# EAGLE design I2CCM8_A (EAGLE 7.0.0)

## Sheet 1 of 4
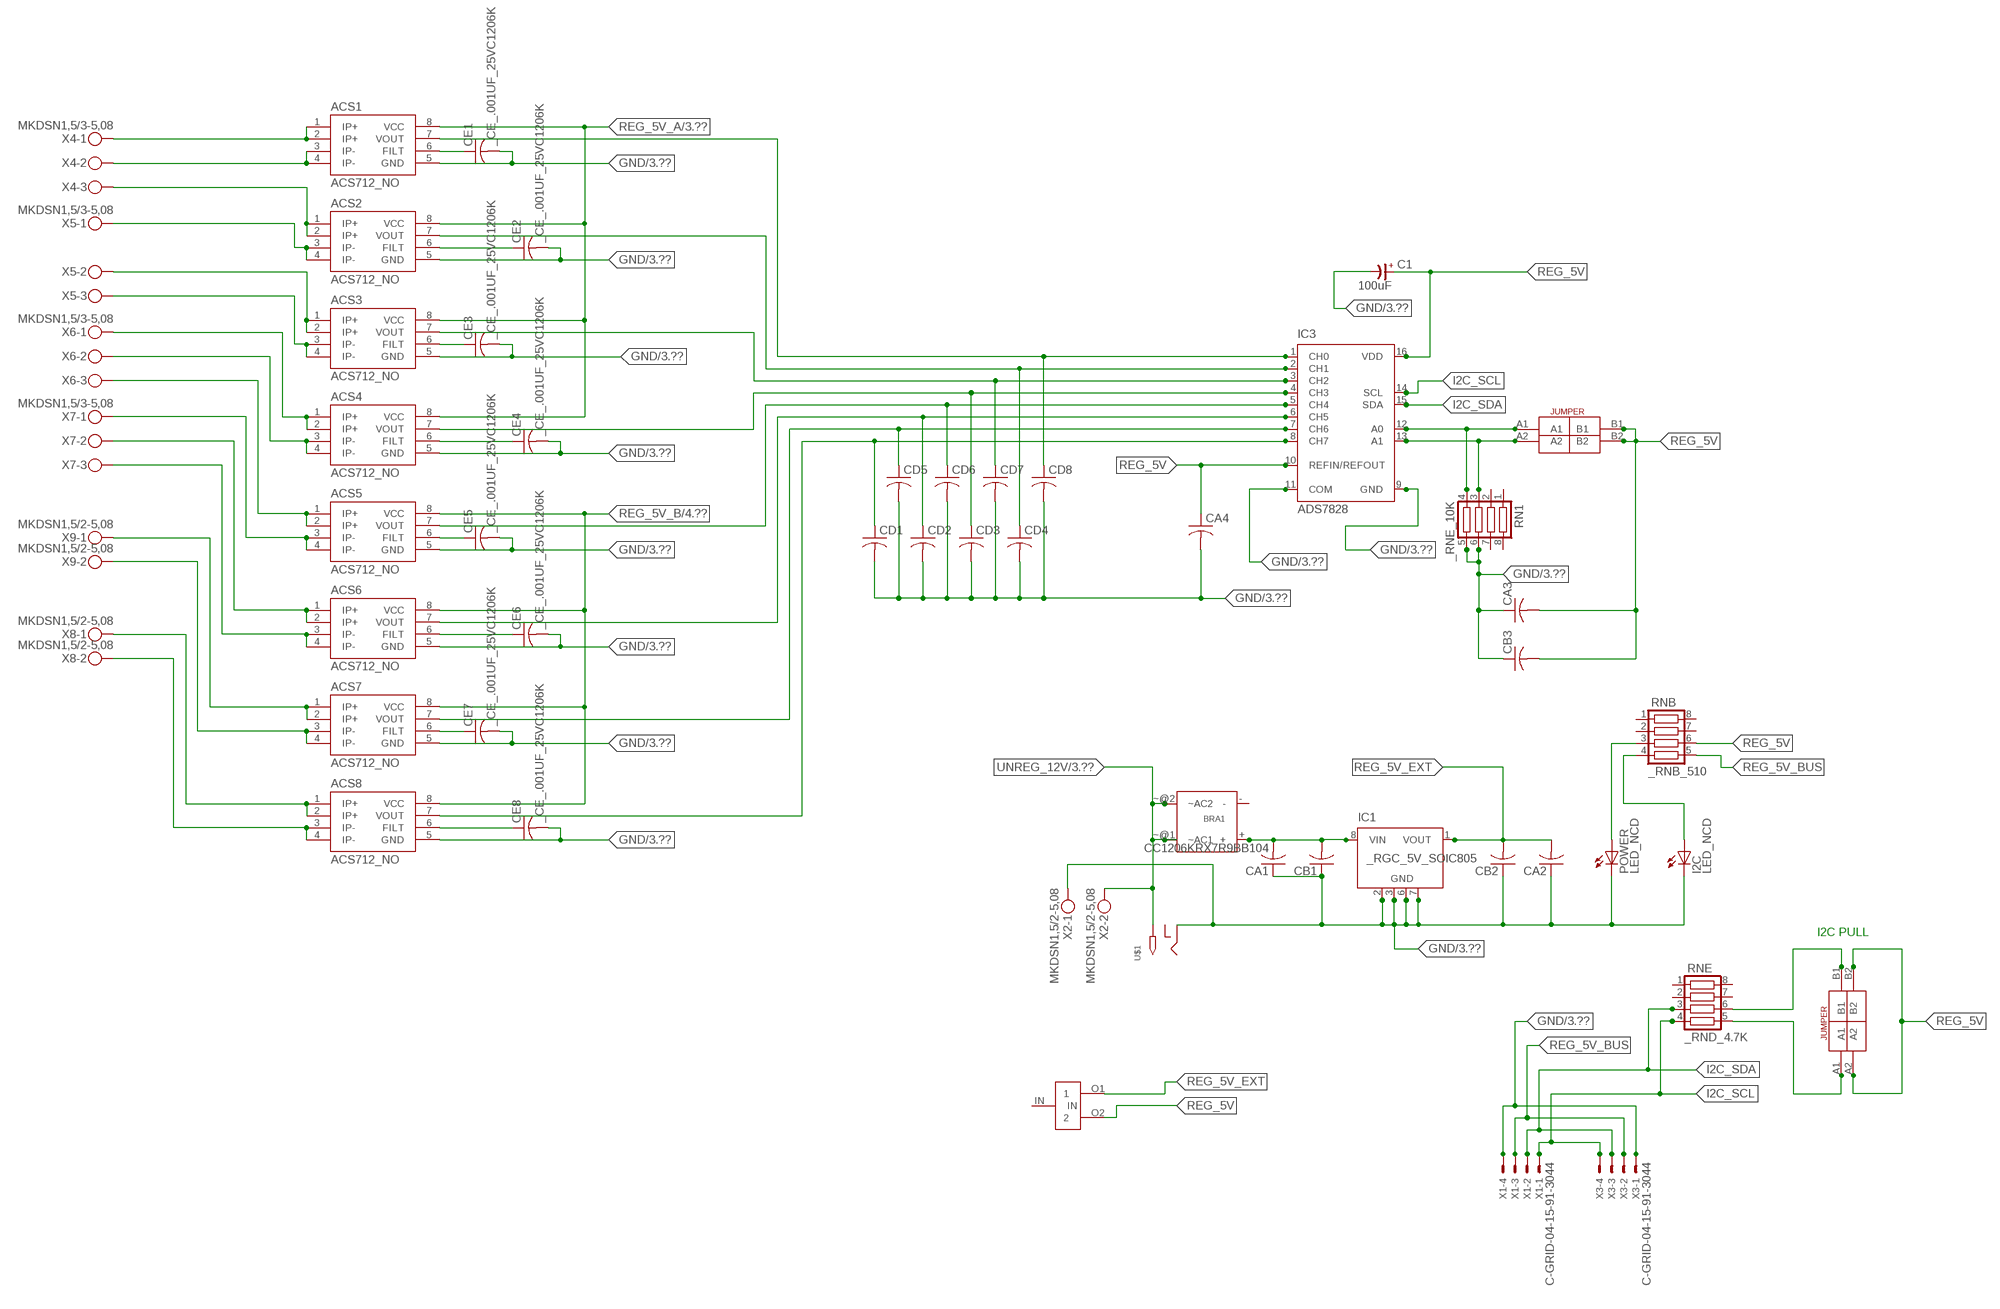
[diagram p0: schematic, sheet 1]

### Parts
ACS1  ACS712_NO  [_MA_DUAL_N-FET]
ACS2  ACS712_NO  [_MA_DUAL_N-FET]
ACS3  ACS712_NO  [_MA_DUAL_N-FET]
ACS4  ACS712_NO  [_MA_DUAL_N-FET]
ACS5  ACS712_NO  [_MA_DUAL_N-FET]
ACS6  ACS712_NO  [_MA_DUAL_N-FET]
ACS7  ACS712_NO  [_MA_DUAL_N-FET]
ACS8  ACS712_NO  [_MA_DUAL_N-FET]
BRA1  MB2S_  [MB2S]
C1  100uF  CP-E-025X060  [E-025X060]
CA1  CC1206KRX7R9BB104  [.1UF]
CA2  CC1206KRX7R9BB104C1206K  [CC1206KRX7R9BB104]
CA3  CC1206KRX7R9BB104C1206K  [CC1206KRX7R9BB104]
CA4  CC1206KRX7R9BB104C1206K  [CC1206KRX7R9BB104]
CB1  TMK316F106ZL-TC1206K  [TMK316F106ZL-T]
CB2  TMK316F106ZL-TC1206K  [TMK316F106ZL-T]
CB3  TMK316F106ZL-TC1206K  [TMK316F106ZL-T]
CD1  _CD_10NF_50VC1206K  [_CD_10NF_50V]
CD2  _CD_10NF_50VC1206K  [_CD_10NF_50V]
CD3  _CD_10NF_50VC1206K  [_CD_10NF_50V]
CD4  _CD_10NF_50VC1206K  [_CD_10NF_50V]
CD5  _CD_10NF_50VC1206K  [_CD_10NF_50V]
CD6  _CD_10NF_50VC1206K  [_CD_10NF_50V]
CD7  _CD_10NF_50VC1206K  [_CD_10NF_50V]
CD8  _CD_10NF_50VC1206K  [_CD_10NF_50V]
CE1  _CE_.001UF_25VC1206K  [CE]
CE2  _CE_.001UF_25VC1206K  [CE]
CE3  _CE_.001UF_25VC1206K  [CE]
CE4  _CE_.001UF_25VC1206K  [CE]
CE5  _CE_.001UF_25VC1206K  [CE]
CE6  _CE_.001UF_25VC1206K  [CE]
CE7  _CE_.001UF_25VC1206K  [CE]
CE8  _CE_.001UF_25VC1206K  [CE]
I2C  LED_NCD  [CHIPLED_0603]
IC1  _RGC_5V_SOIC805  [_RGC_5V_SOIC8]
IC3  ADS7828  [TSSOP16-PW]
POWER  LED_NCD  [CHIPLED_0603]
RN1  _RNE_10K  [RNE]
RNB  _RNB_510  [RNB]
RNE  _RND_4.7K  [RND]
U$1  2.1MMJACK  [PJ-102A]
U$2  LINK_2  [LINK_2]
U$3  JUMPER_2X2  [JUMPER_2X2]
U$4  JUMPER_2X2  [JUMPER_2X2]
X1  C-GRID-04-15-91-3044  [15-91-04]
X2  MKDSN1,5/2-5,08  [MKDSN1,5/2-5,08]
X3  C-GRID-04-15-91-3044  [15-91-04]
X4  MKDSN1,5/3-5,08  [MKDSN1,5/3-5,08]
X5  MKDSN1,5/3-5,08  [MKDSN1,5/3-5,08]
X6  MKDSN1,5/3-5,08  [MKDSN1,5/3-5,08]
X7  MKDSN1,5/3-5,08  [MKDSN1,5/3-5,08]
X8  MKDSN1,5/2-5,08  [MKDSN1,5/2-5,08]
X9  MKDSN1,5/2-5,08  [MKDSN1,5/2-5,08]

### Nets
GND: ACS1.5(GND) ACS2.5(GND) ACS3.5(GND) ACS4.5(GND) ACS5.5(GND) ACS6.5(GND) ACS7.5(GND) ACS8.5(GND) C1.- CA1.1 CA2.1 CA3.1 CA4.2 CB1.1 CB2.1 CB3.1 CD1.2 CD2.2 CD3.2 CD4.2 CD5.2 CD6.2 CD7.2 CD8.2 CE1.2 CE2.2 CE3.2 CE4.2 CE5.2 CE6.2 CE7.2 CE8.2 I2C.C IC1.2(GND) IC1.3(GND) IC1.6(GND) IC1.7(GND) IC3.9(GND) IC3.11(COM) POWER.C RN1.5 RN1.6 U$1.RING X1.4 X2.1 X3.1 ; also sheet 3,4
I2C_SCL: IC3.14(SCL) RNE.4 X1.1 X3.4
I2C_SDA: IC3.15(SDA) RNE.3 X1.2 X3.3
N$1: BRA1.+ CA1.2 CB1.2 IC1.8(VIN)
N$2: POWER.A RNB.3
N$3: I2C.A RNB.4
N$4: RNE.5 U$3.A1
N$5: RNE.6 U$3.B1
N$6: ACS5.7(VOUT) CD6.1 IC3.5(CH4)
N$7: ACS1.1(IP+) ACS1.2(IP+) X4.1
N$8: ACS1.3(IP-) ACS1.4(IP-) X4.2
N$9: ACS1.7(VOUT) CD8.1 IC3.1(CH0)
N$10: ACS2.7(VOUT) CD4.1 IC3.2(CH1)
N$11: ACS3.7(VOUT) CD7.1 IC3.3(CH2)
N$12: ACS4.7(VOUT) CD3.1 IC3.4(CH3)
N$13: ACS2.1(IP+) ACS2.2(IP+) X4.3
N$14: ACS6.7(VOUT) CD2.1 IC3.6(CH5)
N$15: ACS7.7(VOUT) CD5.1 IC3.7(CH6)
N$16: ACS2.3(IP-) ACS2.4(IP-) X5.1
N$17: IC3.12(A0) RN1.4 U$4.A1
N$18: IC3.13(A1) RN1.3 U$4.A2
N$19: ACS3.1(IP+) ACS3.2(IP+) X5.2
N$20: ACS3.3(IP-) ACS3.4(IP-) X5.3
N$21: ACS4.1(IP+) ACS4.2(IP+) X6.1
N$22: ACS4.3(IP-) ACS4.4(IP-) X6.2
N$23: ACS5.1(IP+) ACS5.2(IP+) X6.3
N$24: ACS5.3(IP-) ACS5.4(IP-) X7.1
N$25: ACS6.1(IP+) ACS6.2(IP+) X7.2
N$26: ACS6.3(IP-) ACS6.4(IP-) X7.3
N$27: ACS7.1(IP+) ACS7.2(IP+) X9.1
N$28: ACS7.3(IP-) ACS7.4(IP-) X9.2
N$29: ACS8.1(IP+) ACS8.2(IP+) X8.1
N$30: ACS8.3(IP-) ACS8.4(IP-) X8.2
N$33: ACS1.6(FILT) CE1.1
N$34: ACS2.6(FILT) CE2.1
N$35: ACS3.6(FILT) CE3.1
N$36: ACS4.6(FILT) CE4.1
N$37: ACS8.7(VOUT) CD1.1 IC3.8(CH7)
N$38: ACS5.6(FILT) CE5.1
N$39: ACS6.6(FILT) CE6.1
N$40: ACS7.6(FILT) CE7.1
N$41: ACS8.6(FILT) CE8.1
REG_5V: C1.+ CA3.2 CA4.1 CB3.2 IC3.10(REFIN/REFOUT) IC3.16(VDD) RNB.6 U$2.O2 U$3.A2 U$3.B2 U$4.B1 U$4.B2
REG_5V_A: ACS1.8(VCC) ACS2.8(VCC) ACS3.8(VCC) ACS4.8(VCC) ; also sheet 3
REG_5V_B: ACS5.8(VCC) ACS6.8(VCC) ACS7.8(VCC) ACS8.8(VCC) ; also sheet 4
REG_5V_BUS: RNB.5 X1.3 X3.2
REG_5V_EXT: CA2.2 CB2.2 IC1.1(VOUT) U$2.O1
UNREG_12V: BRA1.~@1(~AC1) BRA1.~@2(~AC2) U$1.TIP X2.2 ; also sheet 3,4
Unconnected: BRA1.- IC1.4(NC) IC1.5(NC) RN1.1 RN1.2 RN1.7 RN1.8 RNB.1 RNB.2 RNB.7 RNB.8 RNE.1 RNE.2 RNE.7 RNE.8 U$1.RING_SW U$2.IN

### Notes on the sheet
- I2C PULL

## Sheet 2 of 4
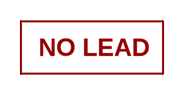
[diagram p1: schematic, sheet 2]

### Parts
U$16  NOPB_LOGO_SYM  [NOPB_LOGO_SYM]

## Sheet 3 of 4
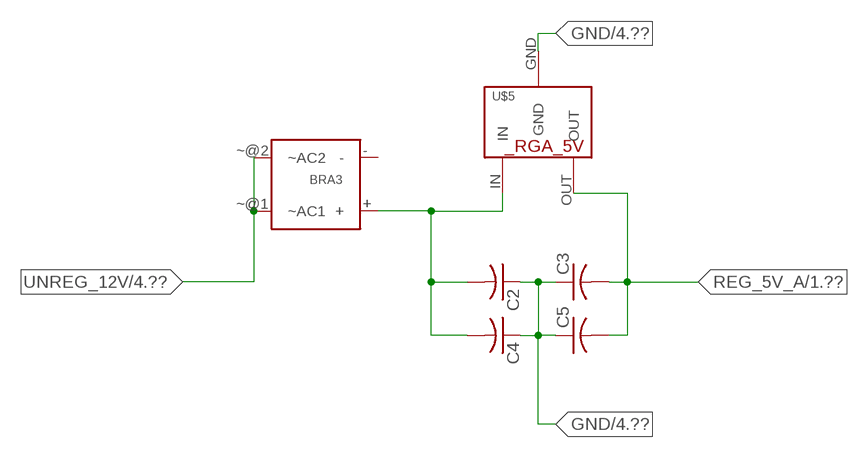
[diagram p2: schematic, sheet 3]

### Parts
BRA3  MB2S_  [MB2S]
C2  _CA_.10UF_50VC1206K  [_CA_.1UF_50V]
C3  _CA_.10UF_50VC1206K  [_CA_.1UF_50V]
C4  _CB_10UF_25VC1206K  [_CB_10UF_25V]
C5  _CB_10UF_25VC1206K  [_CB_10UF_25V]
U$5  _RGA_5V  [_RGA_5V]

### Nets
GND: C2.1 C3.1 C4.1 C5.1 U$5.GND ; also sheet 1,4
N$31: BRA3.+ C2.2 C4.2 U$5.IN
REG_5V_A: C3.2 C5.2 U$5.OUT ; also sheet 1
UNREG_12V: BRA3.~@1(~AC1) BRA3.~@2(~AC2) ; also sheet 1,4
Unconnected: BRA3.-

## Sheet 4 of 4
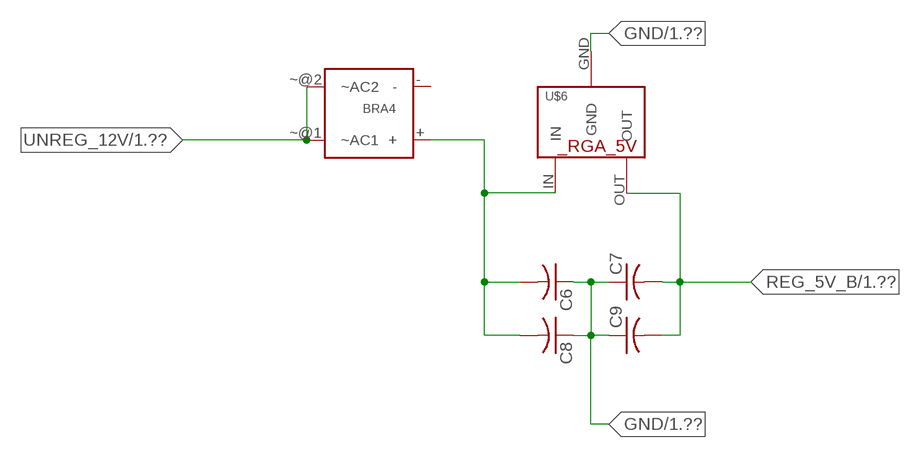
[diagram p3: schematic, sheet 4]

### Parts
BRA4  MB2S_  [MB2S]
C6  _CA_.10UF_50VC1206K  [_CA_.1UF_50V]
C7  _CA_.10UF_50VC1206K  [_CA_.1UF_50V]
C8  _CB_10UF_25VC1206K  [_CB_10UF_25V]
C9  _CB_10UF_25VC1206K  [_CB_10UF_25V]
U$6  _RGA_5V  [_RGA_5V]

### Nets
GND: C6.1 C7.1 C8.1 C9.1 U$6.GND ; also sheet 1,3
N$32: BRA4.+ C6.2 C8.2 U$6.IN
REG_5V_B: C7.2 C9.2 U$6.OUT ; also sheet 1
UNREG_12V: BRA4.~@1(~AC1) BRA4.~@2(~AC2) ; also sheet 1,3
Unconnected: BRA4.-

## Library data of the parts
ACS1-ACS8 = NCD_ULTIMATE_LIBRARY:ACS712_NO: Semiconductor Sensor Current Hall-effect-based isolated linear current sensor Digikey 620-1190-2-ND/ACS712ELCTR-20A-T
BRA1 BRA3 BRA4 = NCD_ULTIMATE_LIBRARY:MB2S: Bridge Rectifier BRA MB2S 200V 500ma Digikey MB2S-TPMSTR-ND/MB2S-TP
C1 = NCD_ULTIMATE_LIBRARY:CP-: Capacitors All Kinds POLARIZED CAP
C2 C3 C6 C7 = NCD_ULTIMATE_LIBRARY:_CA_.10UF_50V: Capacitor .1uF SMT
C4 C5 C8 C9 = NCD_ULTIMATE_LIBRARY:_CB_10UF_25V: Capacitor 10uF SMT
CA1-CA4 = NCD_ULTIMATE_LIBRARY:CC1206KRX7R9BB104: Capacitor CA .1uF 50V SMT C1206K CC1206KRX7R9BB104
CB1-CB3 = NCD_ULTIMATE_LIBRARY:TMK316F106ZL-T: Capacitor CB 10uF SMT 1206 TMK316F106ZL-T
CD1-CD8 = NCD_ULTIMATE_LIBRARY:_CD_10NF_50V: Capacitor 10nF SMT
CE1-CE8 = NCD_ULTIMATE_LIBRARY:_CE_.001UF_25V: Capacitor .001uF SMT
I2C POWER = NCD_ULTIMATE_bhaskar:LED_NCD
IC1 = NCD_ULTIMATE_LIBRARY:_RGC_5V_SOIC8: Regulator Linear 5V Chip Positive VOLTAGE REGULATOR Digikey 497-7267-2-ND/L78L05CD13TR
IC3 = NCD_ULTIMATE_LIBRARY:ADS7828: Semiconductor ADC I2C 12-Bit, 8-Channel Sampling ANALOG-TO-DIGITAL CONVERTER Digikey 296-12402-2-ND Source: www.ti.com .. ADS7828.pdf / ADS7828E/250; MF: TEXAS INSTRUMENTS; MPN: ADS7828E/250; OC_FARNELL: 1470338; OC_NEWARK: 74C7158
RN1 = NCD_ULTIMATE_LIBRARY:_RNE_10K: Resistor Array RNE SMT 10K x 4 Single Resistor Source: http://www.ctscorp.com/components/Datasheets/CTSChipArrayDs.pdf Digikey 742C083103JPTR-ND/742C083103JP; OC_FARNELL: unknown; OC_NEWARK: unknown
RNB = NCD_ULTIMATE_LIBRARY:_RNB_510: Resistor Array RNB SMT 510 x 4 Single Resistor Source: http://www.ctscorp.com/components/Datasheets/CTSChipArrayDs.pdf Digikey 742C083511JPTR-ND/ 742C083511JP; OC_FARNELL: unknown; OC_NEWARK: unknown
RNE = NCD_ULTIMATE_LIBRARY:_RND_4.7K: Resistor Array RND SMT 4.7K x 4 Single Resistor Source: http://www.ctscorp.com/components/Datasheets/CTSChipArrayDs.pdf Digikey 742C083472JPTR-ND/742C083472JP; OC_FARNELL: unknown; OC_NEWARK: unknown
U$1 = NCD_ULTIMATE_CONNECTORS:2.1MMJACK: 2.1mm x 5.5mm DC jack with internal switch. Digikey part #PJ-102A, 4UCON part #05537 By microbuilder.eu
U$2 = NCD_ULTIMATE_LIBRARY:LINK_2: PAD_top
U$3 U$4 = NCD_ULTIMATE_CONNECTORS:JUMPER_2X2
U$5 U$6 = NCD_ULTIMATE_LIBRARY:_RGA_5V: Regulator Linear 5V Digikey 497-7255-2-ND/ L7805CDT-TR
U$16 = PatternAgents-Logos:NOPB_LOGO_SYM: NOPB_LOGO_SYM
X1 X3 = NCD_ULTIMATE_CONNECTORS:C-GRID-04: CONNECTOR 4-Pos I2C wire to board 2.54 mm (0.100") pitch header Digikey WM1342-ND/0015912045; OC_FARNELL: unknown; OC_NEWARK: unknown
X2 X8 X9 = NCD_ULTIMATE_CONNECTORS:MKDSN1,5/2-5,08: MKDSN 1,5/ 2-5,08 Printklemme
X4-X7 = NCD_ULTIMATE_CONNECTORS:MKDSN1,5/3-5,08: MKDSN 1,5/ 3-5,08 Printklemme Nennstrom: 13,5 A Nennspannung: 250 V Rastermaß: 5,08 mm Polzahl: 3 Anschlussart: Schraubanschluss Montage: Löten Anschlussrichtung Leiter/Platine: 0 ° Artikelnummer: 1729131 Source: http://eshop.phoenixcontact.com .. 1729131.pdf

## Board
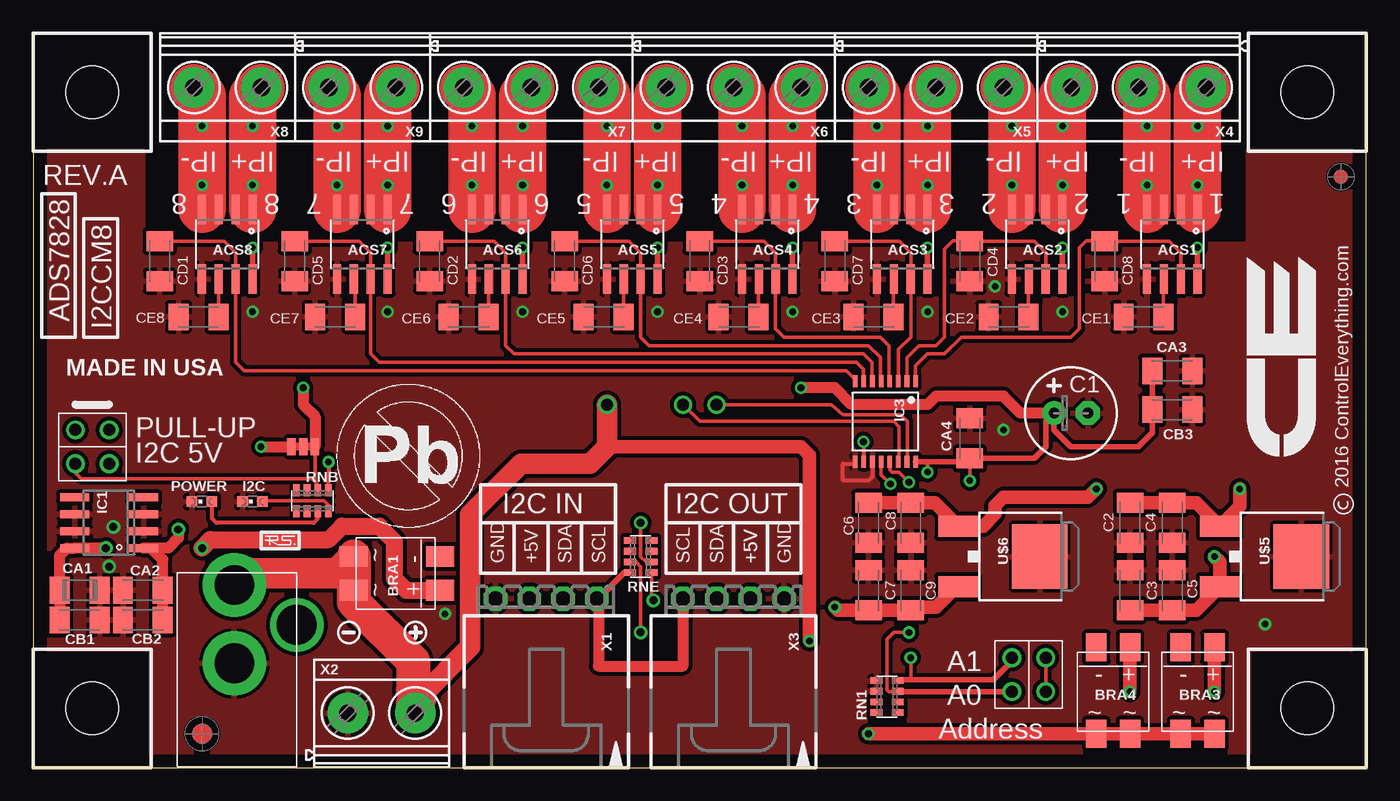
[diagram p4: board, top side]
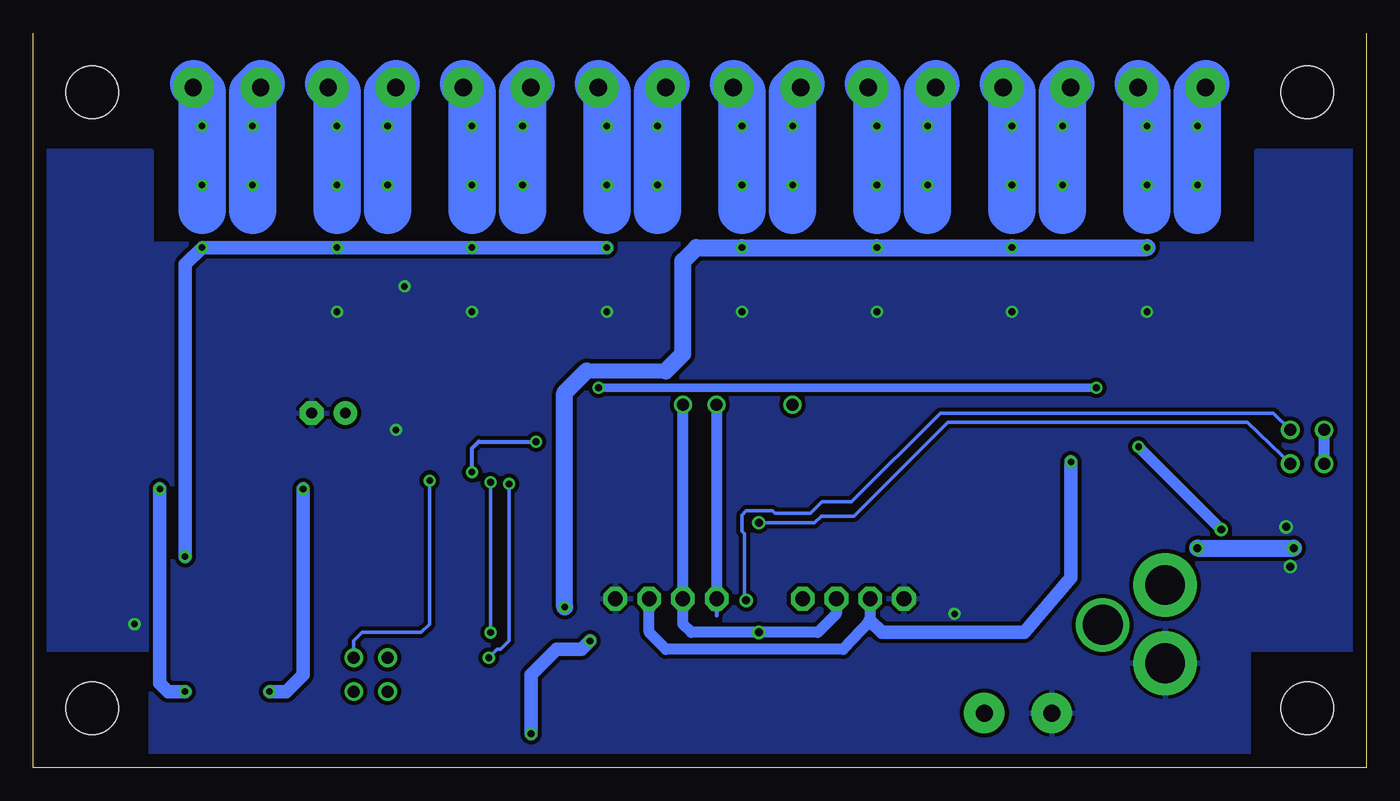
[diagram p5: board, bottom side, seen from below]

Size 100.33 x 55.24 mm. Coordinates in mm from the lower left corner, seen from the top.
Outline: 99.06,0 0,0 0,53.98
Outline: 99.06,0 100.31,0
Outline: 0,54.91 0,53.98
Outline: 99.06,0 100.33,0 100.33,55.24
Outline: 0,55.24 0,53.98
Copper layers (1*16): Top 0.035mm / dielectric 1.5mm / Bottom 0.035mm
Design rules "default": minimum track width 10mil, minimum drill 24mil, track to track 8mil, track to pad 8mil, pad to pad 8mil, via to via 8mil, smd to smd 8mil, copper to edge 40mil, drill to drill 8mil, minimum pad ring 10mil, minimum via ring 8mil, stop-mask expansion 4mil, vias tented up to drill 0mil, thermal gap 10mil
Holes 3.96 mm at 4.45,4.45 95.89,4.45 95.89,50.8 4.45,50.8

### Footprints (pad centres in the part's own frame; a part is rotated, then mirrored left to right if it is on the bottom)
_MA_DUAL_N-FET = smd 0.61 x 2.21: 1 -1.905,-2.616; 2 -0.635,-2.616; 3 0.635,-2.616; 4 1.905,-2.616; 5 1.905,2.616; 6 0.635,2.616; 7 -0.635,2.616; 8 -1.905,2.616
MB2S = smd 1.55 x 2.1: + 0,-6.5; - 2.54,-6.5; ~@1 0,0; ~@2 2.54,0
E-025X060 = drill 0.813 pad 1.778: + -1.27,0 | drill 0.813 pad 1.778 octagon: - 1.27,0
_CA_.1UF_50V = smd 1.5 x 2: 1 -1.5,0; 2 1.5,0
_CB_10UF_25V = smd 1.5 x 2: 1 -1.5,0; 2 1.5,0
.1UF = smd 1.5 x 2: 1 -1.5,0; 2 1.5,0
CC1206KRX7R9BB104 = smd 1.5 x 2: 1 -1.5,0; 2 1.5,0
TMK316F106ZL-T = smd 1.5 x 2: 1 -1.5,0; 2 1.5,0
_CD_10NF_50V = smd 1.5 x 2: 1 -1.5,0; 2 1.5,0
CE = smd 1.5 x 2: 1 -1.5,0; 2 1.5,0
CHIPLED_0603 = smd 0.8 x 0.8: A 0,-0.75; C 0,0.75
_RGC_5V_SOIC8 = smd 0.6 x 2.2: 1 -1.905,-2.6; 2 -0.635,-2.6; 3 0.635,-2.6; 4 1.905,-2.6; 5 1.905,2.6; 6 0.635,2.6; 7 -0.635,2.6; 8 -1.905,2.6
TSSOP16-PW = smd 0.35 x 0.9: 1 -2.275,-3.025; 2 -1.625,-3.025; 3 -0.975,-3.025; 4 -0.325,-3.025; 5 0.325,-3.025; 6 0.975,-3.025; 7 1.625,-3.025; 8 2.275,-3.025; 9 2.275,3.025; 10 1.625,3.025; 11 0.975,3.025; 12 0.325,3.025; 13 -0.325,3.025; 14 -0.975,3.025; 15 -1.625,3.025; 16 -2.275,3.025
RNE = smd 0.5 x 0.9: 1 -1.2,-0.8; 2 -0.4,-0.8; 3 0.4,-0.8; 4 1.2,-0.8; 5 1.2,0.8; 6 0.4,0.8; 7 -0.4,0.8; 8 -1.2,0.8
RNB = smd 0.5 x 0.9: 1 -1.2,-0.8; 2 -0.4,-0.8; 3 0.4,-0.8; 4 1.2,-0.8; 5 1.2,0.8; 6 0.4,0.8; 7 -0.4,0.8; 8 -1.2,0.8
RND = smd 0.5 x 0.9: 1 -1.2,-0.8; 2 -0.4,-0.8; 3 0.4,-0.8; 4 1.2,-0.8; 5 1.2,0.8; 6 0.4,0.8; 7 -0.4,0.8; 8 -1.2,0.8
PJ-102A = drill 3 pad 4.8: RING 0.1,-3.39; TIP 0.1,-9.29 | drill 3 pad 3.251: RING_SW -4.6,-6.29
LINK_2 = smd 1.27 x 0.635: IN 0,0; O1 0,0.889; O2 0,-0.889
JUMPER_2X2 = drill 0.9: A1 0,2.54; A2 0,0; B1 2.54,2.54; B2 2.54,0
_RGA_5V = smd 4.826 x 4.191: GND 0,2.096 | smd 1.6 x 3: IN -2.28,-4.04; OUT 2.28,-4.04
15-91-04 = drill 1.1 pad 1.778 octagon: 1 -3.81,-7.62; 2 -1.27,-7.62; 3 1.27,-7.62; 4 3.81,-7.62
MKDSN1,5/2-5,08 = drill 1.3 pad 3.048: 1 -2.561,0.025; 2 2.519,0.025
MKDSN1,5/3-5,08 = drill 1.3 pad 3.048: 1 -7.641,0.025; 2 -2.561,0.025; 3 2.519,0.025

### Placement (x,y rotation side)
ACS1  85.72,39.37 180 top
ACS2  75.56,39.37 180 top
ACS3  65.41,39.37 180 top
ACS4  55.24,39.37 180 top
ACS5  45.09,39.37 180 top
ACS6  34.92,39.37 180 top
ACS7  24.77,39.37 180 top
ACS8  14.61,39.37 180 top
BRA1  24.13,13.34 90 top
BRA3  88.9,2.54 180 top
BRA4  82.55,2.54 180 top
C1  78.11,26.67 0 top
C2  82.55,18.41 90 top
C3  82.55,13.34 270 top
C4  85.72,18.41 90 top
C5  85.72,13.34 270 top
C6  62.87,18.41 90 top
C7  62.87,13.34 270 top
C8  66.04,18.41 90 top
C9  66.04,13.34 270 top
CA1  3.49,13.34 180 top
CA2  8.26,13.34 0 top
CA3  85.72,29.84 180 top
CA4  70.48,24.77 90 top
CB1  3.49,11.11 180 top
CB2  8.26,11.11 0 top
CB3  85.72,26.92 180 top
CD1  9.53,38.1 270 top
CD2  29.84,38.1 270 top
CD3  50.16,38.1 270 top
CD4  70.48,38.1 270 top
CD5  19.68,38.1 270 top
CD6  40.01,38.1 270 top
CD7  60.33,38.1 270 top
CD8  80.64,38.1 270 top
CE1  83.57,33.91 180 top
CE2  73.41,33.91 180 top
CE3  63.25,33.91 180 top
CE4  53.09,33.91 180 top
CE5  42.93,33.91 180 top
CE6  32.77,33.91 180 top
CE7  22.73,33.91 180 top
CE8  12.45,33.91 180 top
I2C  16.51,20 90 top
IC1  5.71,18.41 90 top
IC3  64.14,26.04 180 top
POWER  12.7,20 90 top
RN1  64.26,5.33 90 top
RNB  21.02,20.07 0 top
RNE  45.72,15.88 270 top
U$1  15.24,4.45 180 top
U$2  20.32,24.13 90 top
U$3  3.17,25.4 270 top
U$4  73.66,5.71 0 top
U$5  93.34,15.88 270 top
U$6  73.66,15.88 270 top
U$10  [VISION_REF15]  12.7,2.54 0 top
U$16  22.63,17.6 0 top
U$19  [VISION_REF10]  98.42,44.45 0 top
U$21  [ICON_USA]  14.35,30.73 180 top
U$22  [ICON_MINUS]  23.75,10.16 180 top
U$24  [ICON_PLUS]  28.77,10.16 90 top
X1  38.61,5.08 180 top
X2  26.23,4.06 0 top
X3  52.7,5.08 180 top
X4  80.64,51.18 180 top
X5  65.41,51.18 180 top
X6  50.16,51.18 180 top
X7  34.92,51.18 180 top
X8  14.61,51.18 180 top
X9  24.77,51.18 180 top

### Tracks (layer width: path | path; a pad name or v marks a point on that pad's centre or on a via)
GND  (via drill 0.5, 0.6)
  Top 0.305: IC3.11 63.16,21.89 62.87,21.59 60.96,21.59 60.96,22.86 61.71,22.86 IC3.9
  Top 0.406: 34.8,12.38 X1.4
  Top 0.61: C4.1 85.72,17.14 | C8.1 66.04,17.14
  Top 0.813: X3.1 56.52,12.06
  other vias: 5.71,15.11 6.03,18.1 72.39,36.2 73.03,25.4 77.47,34.29 67.31,34.29 30.99,11.56 57.15,34.29 46.99,34.29 36.83,34.29 26.67,34.29 16.51,34.29 92.71,10.79
  pour Bottom (isolate 0.305): -0.64,8.89 -0.64,46.35 8.26,46.35 8.26,40.01 8.26,39.37 91.44,39.37 91.44,46.35 100.97,46.35 100.97,40.01 100.97,8.89 91.44,8.89 91.44,-0.64 8.89,-0.64 8.89,8.89
  pour Top (isolate 0.305): -1.91,46.35 8.26,46.35 8.26,39.37 91.44,39.37 91.44,46.35 102.87,46.35 102.87,8.89 91.44,8.89 91.44,-1.91 8.89,-1.91 8.89,8.89 -1.91,8.89
I2C_SCL  (via drill 0.9)
  Top 0.254: v48.9,27.3 50.16,26.04 64.77,26.04 65.15,25.65 65.15,23.05 IC3.14
  Top 0.406: RNE.4 44.51,14.68 42.55,12.7
  Top 0.813: X3.4 48.9,7.62 42.55,7.62 42.55,12.7 X1.1
  Bottom 0.305: 48.9,12.06 48.9,11.43
  Bottom 0.813: v48.9,27.3 X3.4 48.9,12.06
I2C_SDA  (via drill 0.6, 0.9)
  Top 0.254: RNE.3 45.36,15.47 45.72,15.11 v45.72,10.16 | v51.44,27.3 60.07,27.3 60.96,26.54 65.28,26.54 65.79,26.04 65.79,23.04 IC3.15
  Top 0.61: X1.2 39.88,12.38
  Bottom 0.813: 39.88,12.38 39.88,11.56 41.27,10.16 v45.72,10.16 50.8,10.16 51.44,10.79 X3.3 v51.44,27.3
  Bottom 1.016: 39.88,12.38 X1.2
N$1  (via drill 0.6)
  Top 0.813: CB1.2 CA1.2 1.99,15.96 2.54,16.51 IC1.8 v5.46,16.51
  Top 1.27: v12.7,16.51 13.34,17.14 22.23,17.14 23.24,18.16 26.04,18.16 27.18,17.02 27.18,14.22 28.07,13.34 BRA1.+
  Bottom 1.27: v12.7,16.51 v5.46,16.51
N$2
  Top 0.305: RNB.3 21.4,18.95 21.4,18.7 21.12,18.41 13.78,18.41 13.45,18.74 POWER.A
N$3
  Top 0.254: 22.23,18.95 22.23,19.74 21.9,20.07 16.94,20.07
  Top 0.305: RNB.4 22.23,18.95 | 16.94,20.07 I2C.A
N$4  (via drill 0.6)
  Top 0.254: RNE.5 46.52,12.6 v46.67,12.57
  Bottom 0.254: U$3.A1 6.99,26.67 32.07,26.67 38.73,20 40.96,20 41.85,19.11 44.51,19.11 44.7,19.3 46.67,19.3 46.99,18.99 46.99,17.78 46.8,17.59 46.8,12.7 v46.67,12.57
N$5  (via drill 0.6)
  Top 0.254: RNE.6 46.12,15.47 45.72,15.88 v45.72,18.41
  Bottom 0.254: v45.72,18.41 41.53,18.41 41.02,18.92 38.54,18.92 31.5,25.97 8.95,25.97 6.35,23.5 U$3.B1
N$6
  Top 0.254: CD6.1 44.85,39.6 45.72,38.73 ACS5.7 45.72,32.38 46.35,31.75 62.87,31.75 63.75,30.86 63.75,29.12 IC3.5
N$7  (via drill 0.5)
  Top 0.254: ACS1.2 ACS1.1
  Top 3.556: ACS1.1 v87.63,43.81 v87.63,48.26 87.63,50.5 X4.1
  Bottom 3.556: 87.63,41.91 v87.63,43.81 v87.63,48.26 87.63,50.8 88.27,51.44
N$8  (via drill 0.5)
  Top 0.254: ACS1.4 ACS1.3
  Top 3.556: ACS1.4 v83.82,43.81 v83.82,48.26 83.82,50.54 X4.2
  Bottom 3.556: 83.82,41.91 v83.82,43.81 v83.82,48.26 83.82,50.8 83.19,51.44
N$9
  Top 0.254: ACS1.7 86.36,38.73 85.5,39.6 CD8.1 80.62,39.62 79.25,39.62 78.74,39.12 78.74,33.02 78.11,32.38 69.85,32.38 68.58,31.11 67.31,31.11 66.41,30.21 IC3.1
N$10
  Top 0.254: ACS2.7 76.2,38.73 75.33,39.6 CD4.1 70.46,39.62 69.22,39.62 68.58,38.99 68.58,32.38 67.94,31.75 66.67,31.75 65.76,30.84 IC3.2
N$11
  Top 0.254: CD7.1 65.17,39.6 66.04,38.73 ACS3.7 66.04,32.38 65.11,31.45 IC3.3
N$12
  Top 0.254: CD3.1 55.02,39.6 55.88,38.73 ACS4.7 55.88,33.02 56.52,32.38 63.75,32.38 64.39,31.75 64.39,29.13 IC3.4
N$13  (via drill 0.5)
  Top 0.254: ACS2.2 ACS2.1
  Top 3.556: ACS2.1 v77.47,43.81 v77.47,48.26 77.47,50.5 X4.3
  Bottom 3.556: 77.47,41.91 v77.47,43.81 v77.47,48.26 77.47,50.8 78.11,51.44
N$14
  Top 0.254: CD2.1 34.7,39.6 35.56,38.73 ACS6.7 35.56,31.75 36.2,31.11 62.48,31.11 63.12,30.48 63.12,29.1 IC3.6
N$15
  Top 0.254: CD5.1 24.54,39.6 25.4,38.73 ACS7.7 25.4,31.11 26.04,30.48 61.98,30.48 62.48,29.97 62.48,29.09 IC3.7
N$16  (via drill 0.5)
  Top 0.254: ACS2.4 ACS2.3
  Top 3.556: ACS2.4 v73.66,43.81 v73.66,48.26 73.66,50.54 X5.1
  Bottom 3.556: 73.66,41.91 v73.66,43.81 v73.66,48.26 73.66,50.8 73.03,51.44
N$17  (via drill 0.5)
  Top 0.254: IC3.12 63.81,22.03 v64.52,21.34 | v66.04,8.26 66.04,6.6
  Top 0.406: U$4.A1 73.66,8 72.26,6.6 66.04,6.6 65.13,6.6 RN1.4
  Bottom 0.254: v64.52,21.34 64.52,9.53 65.15,8.89 65.41,8.89 v66.04,8.26
N$18  (via drill 0.5)
  Top 0.254: v65.91,10.16 64.77,10.16 64.26,9.65 64.26,5.84 64.39,5.71 65.04,5.71 RN1.3 | IC3.13 64.46,22.41 64.64,22.23 65.15,22.23 v65.91,21.46
  Top 0.406: U$4.A2 65.08,5.71 RN1.3
  Bottom 0.254: v65.91,21.46 v65.91,10.16
N$19  (via drill 0.5)
  Top 0.254: ACS3.2 ACS3.1
  Top 3.556: ACS3.1 v67.31,43.81 v67.31,48.26 67.31,50.5 X5.2
  Bottom 3.556: 67.31,41.91 v67.31,43.81 v67.31,48.26 67.31,50.8 67.94,51.44
N$20  (via drill 0.5)
  Top 0.254: ACS3.4 ACS3.3
  Top 3.556: ACS3.4 v63.5,43.81 v63.5,48.26 63.5,50.54 X5.3
  Bottom 3.556: 63.5,41.91 v63.5,43.81 v63.5,48.26 63.5,50.8 62.87,51.44
N$21  (via drill 0.5)
  Top 0.254: ACS4.2 ACS4.1
  Top 3.556: ACS4.1 v57.15,43.81 v57.15,48.26 57.15,50.5 X6.1
  Bottom 3.556: 57.15,41.91 v57.15,43.81 v57.15,48.26 57.15,50.8 57.78,51.44
N$22  (via drill 0.5)
  Top 0.254: ACS4.4 ACS4.3
  Top 3.556: ACS4.4 v53.34,43.81 v53.34,48.26 53.34,50.54 X6.2
  Bottom 3.556: 53.34,41.91 v53.34,43.81 v53.34,48.26 53.34,50.8 52.7,51.44
N$23  (via drill 0.5)
  Top 0.254: ACS5.2 ACS5.1
  Top 3.556: ACS5.1 v46.99,43.81 v46.99,48.26 46.99,50.5 X6.3
  Bottom 3.556: 46.99,41.91 v46.99,43.81 v46.99,48.26 46.99,50.8 47.62,51.44
N$24  (via drill 0.5)
  Top 0.254: ACS5.4 ACS5.3
  Top 3.556: ACS5.4 v43.18,43.81 v43.18,48.26 43.18,50.54 X7.1
  Bottom 3.556: 43.18,41.91 v43.18,43.81 v43.18,48.26 43.18,50.8 42.55,51.44
N$25  (via drill 0.5)
  Top 0.254: ACS6.2 ACS6.1
  Top 3.556: ACS6.1 v36.83,43.81 v36.83,48.26 36.83,50.5 X7.2
  Bottom 3.556: 36.83,41.91 v36.83,43.81 v36.83,48.26 36.83,50.8 37.47,51.44
N$26  (via drill 0.5)
  Top 0.254: ACS6.4 ACS6.3
  Top 3.556: ACS6.4 v33.02,43.81 v33.02,48.26 33.02,50.54 X7.3
  Bottom 3.556: 33.02,41.91 v33.02,43.81 v33.02,48.26 33.02,50.8 32.38,51.44
N$27  (via drill 0.5)
  Top 0.254: ACS7.2 ACS7.1
  Top 3.556: ACS7.1 v26.67,43.81 v26.67,48.26 26.67,50.5 X9.1
  Bottom 3.556: 26.67,41.91 v26.67,43.81 v26.67,48.26 26.67,50.8 27.3,51.44
N$28  (via drill 0.5)
  Top 0.254: ACS7.4 ACS7.3
  Top 3.556: ACS7.4 v22.86,43.81 v22.86,48.26 22.86,50.54 X9.2
  Bottom 3.556: 22.86,41.91 v22.86,43.81 v22.86,48.26 22.86,50.8 22.23,51.44
N$29  (via drill 0.5)
  Top 0.254: ACS8.2 ACS8.1
  Top 3.556: ACS8.1 v16.51,43.81 v16.51,48.26 16.51,50.5 X8.1
  Bottom 3.556: 17.14,51.44 16.51,50.8 v16.51,48.26 v16.51,43.81 16.51,41.91
N$30  (via drill 0.5)
  Top 0.254: ACS8.4 ACS8.3
  Top 3.556: ACS8.4 v12.7,43.81 v12.7,48.26 12.7,50.54 X8.2
  Bottom 3.556: 12.06,51.44 12.7,50.8 v12.7,48.26 v12.7,43.81 12.7,41.91
N$31  (via drill 0.5)
  Top 1.016: C2.2 C4.2 87.55,19.91 U$5.IN 90.81,19.66 v90.81,20.95 | BRA3.+ v88.9,5.71
  Bottom 1.016: v88.9,5.71 90.17,5.71 90.81,6.35 v90.81,20.95
N$32  (via drill 0.5)
  Top 1.016: C6.2 C8.2 67.86,19.91 U$6.IN 71.5,18.16 72.39,19.05 72.39,19.68 73.03,20.32 79.38,20.32 v80.01,20.95 | v82.55,5.71 BRA4.+
  Bottom 1.016: v80.01,20.95 80.01,6.99 81.28,5.71 v82.55,5.71
N$33
  Top 0.254: CE1.1 85.07,36.73 ACS1.6
N$34
  Top 0.254: CE2.1 74.91,36.73 ACS2.6
N$35
  Top 0.254: CE3.1 64.75,36.73 ACS3.6
N$36
  Top 0.254: CE4.1 54.59,36.73 ACS4.6
N$37
  Top 0.254: CD1.1 14.38,39.6 15.24,38.73 ACS8.7 15.24,30.48 15.88,29.84 61.21,29.84 61.85,29.21 61.85,29.07 IC3.8
N$38
  Top 0.254: CE5.1 44.43,36.73 ACS5.6
N$39
  Top 0.254: CE6.1 34.27,36.73 ACS6.6
N$40
  Top 0.254: CE7.1 24.23,36.65 ACS7.6
N$41
  Top 0.254: CE8.1 13.95,36.73 ACS8.6
REG_5V  (via drill 0.5)
  Top 0.254: RNB.6 21.42,21.29 21.21,21.5 | 21.21,21.5 20.99,21.72 3.62,21.72 3.17,22.16 U$3.B2 | U$4.B2 U$4.B1 | v70.48,21.59 CA4.1 | U$2.O2 21.21,21.5
  Top 0.305: IC3.16 67.16,23.01 67.31,22.86 v67.31,22.23 | v62.48,24.51 62.48,23.04 IC3.10
  Top 0.406: IC3.16 70.23,23.01 CA4.1 75.33,23.27 76.2,24.13 76.2,26.04 C1.+ 76.83,25.4 78.11,24.13 83.19,24.13 84.22,25.17 CB3.2 CA3.2
  Top 0.813: C1.+ 74.3,26.67 73.03,27.94 67.94,27.94 67.31,27.3 61.59,27.3 60.33,28.57 v57.78,28.57 | v20.32,28.57 20.32,27.3 21.21,26.42 U$2.O2
  Bottom 0.254: U$4.B1 76.2,9.53 75.56,10.16 71.12,10.16 70.48,10.79 v70.48,21.59
  Bottom 0.305: v67.31,22.23 67.31,24 66.8,24.51 v62.48,24.51
  Bottom 0.635: v57.78,28.57 v20.32,28.57
  Bottom 0.813: U$3.B2 U$3.A2
REG_5V_A  (via drill 0.5)
  Top 0.406: ACS1.8 v87.63,39.12 | ACS2.8 v77.47,39.12 | ACS3.8 v67.31,39.12 | ACS4.8 v57.15,39.12
  Top 1.016: C3.2 C5.2 87.55,11.84 U$5.OUT 89.31,15.47 v88.9,15.88
  Bottom 1.016: v88.9,15.88 88.9,37.85 v87.63,39.12 v77.47,39.12 v67.31,39.12 v57.15,39.12
REG_5V_B  (via drill 0.5)
  Top 0.406: ACS5.8 v46.99,39.12 | ACS6.8 v36.83,39.12 | ACS7.8 v26.67,39.12 | ACS8.8 v16.51,39.12
  Top 1.016: U$6.OUT 69.47,13.6 67.94,12.06 66.27,12.06 C9.2 C7.2 60.55,11.84 v60.33,12.06
  Bottom 1.143: 58.67,29.84 52.7,29.84
  Bottom 1.27: v60.33,12.06 60.33,28.19 58.67,29.84 | 52.7,29.84 51.44,31.11 51.44,38.1 50.42,39.12 v46.99,39.12 v36.83,39.12 v26.67,39.12 v16.51,39.12
REG_5V_BUS  (via drill 0.5)
  Top 0.305: RNB.5 22.26,22.9 v22.23,22.99
  Top 0.61: X1.3 37.34,12.38 | X3.2 53.98,12.06
  Bottom 0.813: 37.34,12.38 37.34,11.05 39.37,8.89 52.7,8.89 53.98,10.16 53.98,12.06
  Bottom 1.016: v22.23,22.99 22.23,14.29 25.72,10.16 36.45,10.16 37.34,11.05 | 37.34,12.38 X1.3 | 53.98,12.06 X3.2
REG_5V_EXT  (via drill 0.5, 0.6)
  Top 0.813: CB2.2 CA2.2 9.76,15.64 8.89,16.51 | 8.89,16.51 IC1.1 | v10.92,17.91 10.92,17.27 10.16,16.51 8.89,16.51 | v17.14,24.13 U$2.O1
  Bottom 0.813: v17.14,24.13 v10.92,17.91
UNREG_12V  (via drill 0.5, 0.9)
  Top 1.016: BRA4.~@2 BRA4.~@1 BRA3.~@2 BRA3.~@1 v62.87,2.54 | v58.42,9.53 58.42,23.5 57.78,24.13 43.81,24.13 43.18,24.77
  Top 1.524: v43.18,27.3 43.18,24.77 43.18,24.13 41.91,22.86 36.7,22.86 32.89,19.05 32.89,9.08 29.11,5.3 28.57,4.76
  Top 2.286: BRA1.~@2 22.86,14.61 16.01,14.61
  Top 2.54: 16.01,14.61 U$1.TIP | X2.2 28.55,4.45 28.57,4.76 | BRA1.~@2 BRA1.~@1 24.13,12.45 28.57,8 28.57,5.84 29.11,5.3
  Bottom 1.016: v62.87,2.54 62.87,6.99 60.96,8.89 59.05,8.89 v58.42,9.53

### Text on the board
tNames: IP- | IP+ | IP- | IP+ | IP- | IP+ | IP- | IP+ | IP- | IP+ | IP- | IP+ | IP- | IP+ | IP- | IP+ | REV.A | ADS7828 | 8 | 8 | 7 | 7 | 6 | 6 | 5 | 5 | 4 | 4 | 3 | 3 | 2 | 2 | 1 | 1 | I2CCM8 | PULL-UP | I2C 5V | 2016 ControlEverything.com | I2C IN | I2C OUT | GND | +5V | SDA | SCL | SCL | SDA | +5V | +5V | GND | A1 | A0 | Address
